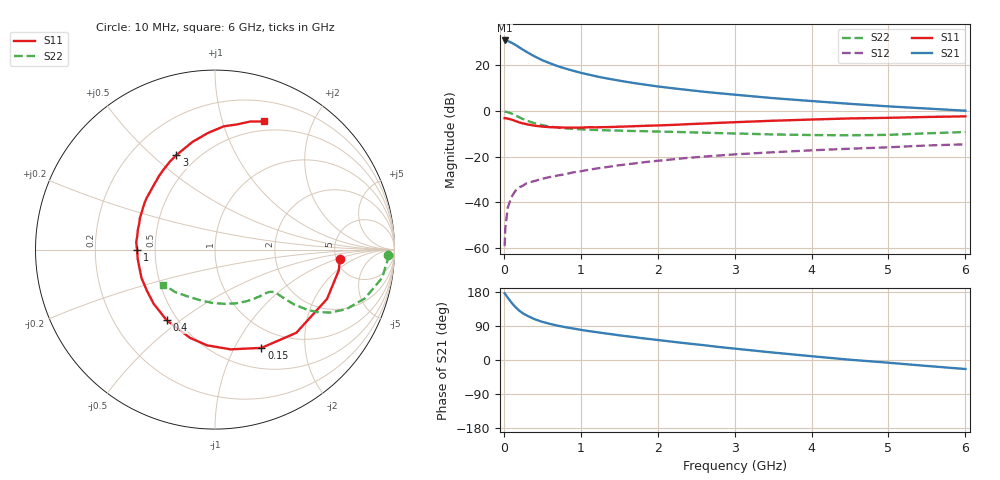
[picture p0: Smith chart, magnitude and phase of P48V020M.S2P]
! SIEMENS Small Signal Semiconductors
! BFP182
! Si NPN RF Bipolar Junction Transistor in SOT143
! VCE = 8 V  IC = 20 mA
! Common Emitter S-Parameters:  March  1996
# GHz  S  MA  R  50
!  f  S11  S21  S12  S22
! GHz  MAG  ANG  MAG  ANG  MAG  ANG  MAG  ANG
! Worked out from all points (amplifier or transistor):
!   36 points, 10 MHz to 6 GHz, reference 50 ohm
!   highest |S21| = 30.9 dB at 10 MHz (marker M1)
!   |S21| within 3 dB of that: start of sweep to 200.2 MHz
!   unconditionally stable (mu >= 1): 928 MHz to 5.539 GHz
!   at 250 MHz: K = 0.45, MSG = 29.7 dB, |S12| = -32.6 dB
!   at 1.4 GHz: K = 1.12, MAG = 17.0 dB, |S12| = -24.3 dB
!   at 6 GHz: K = 0.96, MSG = 7.4 dB, |S12| = -14.6 dB
!   S11 on the Smith chart (normalised r, x): 10 MHz: 5.37, -1.12; 150 MHz: 0.75, -1.29; 400 MHz: 0.44, -0.44; 1 GHz: 0.39, -0.00; 3 GHz: 0.39, +0.60; 6 GHz: 0.40, +1.37
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0.01  0.6975 -4.4  35.02 176.0  0.0011 85.9  0.9649 -1.7
0.02  0.6995 -9.5  34.96 173.7  0.0028 81.1  0.9623 -3.8
0.05  0.682 -23.8  34.04 164.7  0.0076 82.3  0.9441 -9.6
0.1  0.6481 -45.7  31.25 151.2  0.0131 68.4  0.8786 -18.0
0.15  0.6056 -64.7  27.99 139.7  0.0179 61.6  0.8035 -24.4
0.2  0.5625 -81.1  24.81 130.3  0.0212 57.8  0.7301 -28.7
0.25  0.5353 -94.7  21.88 122.9  0.0234 54.8  0.6656 -31.5
0.3  0.5111 -105.8  19.47 117.2  0.0264 52.7  0.6131 -33.1
0.4  0.4767 -124.5  15.69 107.7  0.0294 50.2  0.538 -34.7
0.5  0.4559 -138.6  12.93 100.7  0.0329 49.8  0.4892 -35.1
0.6  0.4428 -149.2  11.1 95.3  0.0359 50.6  0.4558 -35.2
0.7  0.4392 -158.7  9.566 90.6  0.0387 51.3  0.4334 -35.3
0.8  0.433 -166.8  8.502 86.6  0.0414 51.3  0.4176 -35.5
1  0.4339 -179.5  6.853 79.6  0.0479 52.0  0.3974 -36.4
1.1  0.4407 174.6  6.28 76.4  0.0517 52.2  0.39 -37.1
1.6  0.4584 152.9  4.336 62.6  0.0681 50.7  0.3677 -42.5
2.2  0.4967 133.0  3.141 48.0  0.0877 47.2  0.3496 -51.8
3  0.5685 112.3  2.278 30.0  0.1124 40.5  0.3226 -68.0
3.5  0.6127 101.9  1.914 19.7  0.125 35.9  0.3071 -79.8
4.5  0.6883 86.0  1.435 0.7  0.1496 27.3  0.2939 -106.5
5.5  0.7403 74.6  1.133 -15.7  0.1759 19.7  0.3244 -133.1
6  0.7643 69.1  1.015 -23.8  0.1866 14.9  0.347 -145.8
